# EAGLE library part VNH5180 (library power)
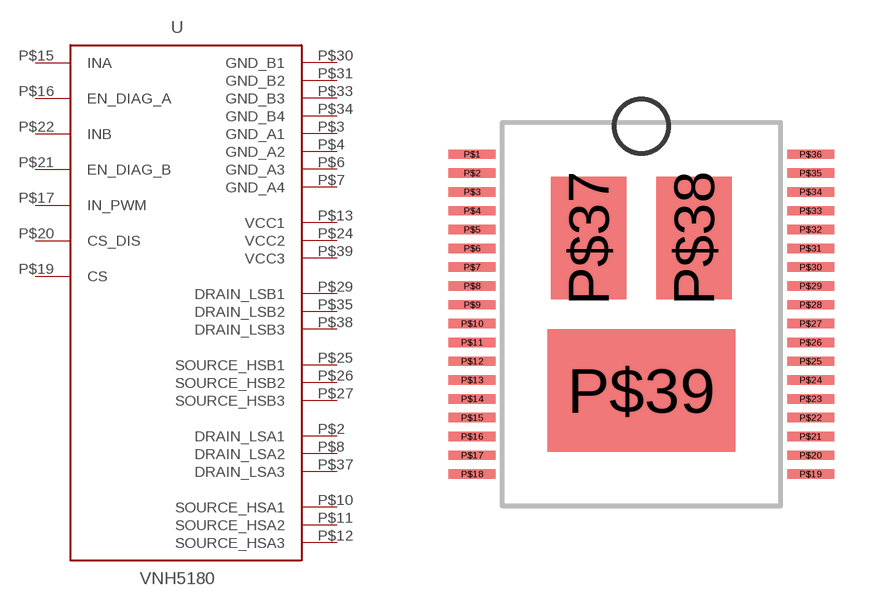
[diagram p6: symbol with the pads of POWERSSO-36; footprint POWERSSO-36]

Designator prefix U

## VNH5180  [POWERSSO-36]
P$2  DRAIN_LSA1
P$3  GND_A1
P$4  GND_A2
P$6  GND_A3
P$7  GND_A4
P$8  DRAIN_LSA2
P$10  SOURCE_HSA1
P$11  SOURCE_HSA2
P$12  SOURCE_HSA3
P$13  VCC1
P$15  INA
P$16  EN_DIAG_A
P$17  IN_PWM
P$19  CS
P$20  CS_DIS
P$21  EN_DIAG_B
P$22  INB
P$24  VCC2
P$25  SOURCE_HSB1
P$26  SOURCE_HSB2
P$27  SOURCE_HSB3
P$29  DRAIN_LSB1
P$30  GND_B1
P$31  GND_B2
P$33  GND_B3
P$34  GND_B4
P$35  DRAIN_LSB2
P$37  DRAIN_LSA3
P$38  DRAIN_LSB3
P$39  VCC3

## Footprint POWERSSO-36 (pad centres in mm)
smd 1.25 x 0.25: P$1 -4.5,4.25; P$2 -4.5,3.75; P$3 -4.5,3.25; P$4 -4.5,2.75; P$5 -4.5,2.25; P$6 -4.5,1.75; P$7 -4.5,1.25; P$8 -4.5,0.75; P$9 -4.5,0.25; P$10 -4.5,-0.25; P$11 -4.5,-0.75; P$12 -4.5,-1.25; P$13 -4.5,-1.75; P$14 -4.5,-2.25; P$15 -4.5,-2.75; P$16 -4.5,-3.25; P$17 -4.5,-3.75; P$18 -4.5,-4.25; P$19 4.5,-4.25; P$20 4.5,-3.75; P$21 4.5,-3.25; P$22 4.5,-2.75; P$23 4.5,-2.25; P$24 4.5,-1.75; P$25 4.5,-1.25; P$26 4.5,-0.75; P$27 4.5,-0.25; P$28 4.5,0.25; P$29 4.5,0.75; P$30 4.5,1.25; P$31 4.5,1.75; P$32 4.5,2.25; P$33 4.5,2.75; P$34 4.5,3.25; P$35 4.5,3.75; P$36 4.5,4.25
smd 2 x 3.25: P$37 -1.4,2.025; P$38 1.4,2.025
smd 5 x 3.25: P$39 0,-2.025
